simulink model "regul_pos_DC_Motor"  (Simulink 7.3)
settings: Solver=ode15s  StartTime=0.0  StopTime=150  RelTol=1e-3
StopFcn:
  | close all, clc
  | load pos_vit.mat
  | plot(x(1,:),x(2,:), x(1,:),x(4,:))
  | grid
  | title('Régulation de vitesse DC Motor')
  | gtext('Consigne)')
  | gtext('Position')
  | xlabel('temps')
  | figure
  | plotyy(x(1,:),x(3,:),x(1,:),x(5,:))
  | title('Position et Signal de commande')
  | gtext('signal de commande')
  | gtext('position linéaire')
  | grid
  | xlabel('temps')
libraries: fl_lib x17, nesl_utility x6, elec_lib x1

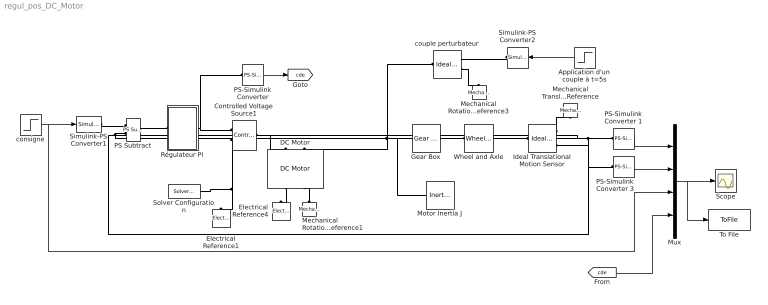
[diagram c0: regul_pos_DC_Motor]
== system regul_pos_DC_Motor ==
  Application d'un couple à t=5s : Step  Time=55  After=-0.5e-3  SampleTime=0
  Controlled Voltage Source1 : fl_lib/Electrical/Electrical Sources/Controlled Voltage Source  DialogController=NetworkEngine.DynNeDlgSource  SystemSampleTime=-1  i_Log=off  v_Log=off  LocalVarNames=|current|voltage|power  LocalVarDescs=|Current (A)|Voltage (V)|Power (W)  LocalVarLogging=[0 0 0]
  DC Motor : elec_lib/Actuators & Drivers/DC Motor  DialogController=NetworkEngine.DynNeDlgSource  SystemSampleTime=-1  parameterization=1  Ra=3.9 Ohm  La=1.2e-05 H  emf_or_torque=1  Kv=7.2e-05 V/rpm  Ki=6.876e-04 N*m/A  T_stall=2.4e-04 N*m  w_max=1.91e+04 rpm  w_rated=1.5e+04 rpm  P_rated=0.08 W  V_rated=1.5 V  J=0.01 g*cm^2  lam=1e-08 N*m/(rad/s)  speed0=0 rpm  current_Log=off  voltage_Log=off  power_Log=off  i2r_Log=off  torque_Log=off  speed_Log=off  LocalVarNames=|current|voltage|power|i2r|torque|speed  LocalVarDescs=|Current (A)|Voltage (V)|Power (W)|Electrical losses (W)|Torque (Nm)|Angular speed (rad/s)  LocalVarLogging=[0 0 0 0 0 0]
  Electrical Reference1 : fl_lib/Electrical/Electrical Elements/Electrical Reference  DialogController=NetworkEngine.DynNeDlgSource  SystemSampleTime=-1  i_Log=off  LocalVarNames=|i  LocalVarDescs=|i  LocalVarLogging=[]
  Electrical Reference4 : fl_lib/Electrical/Electrical Elements/Electrical Reference  DialogController=NetworkEngine.DynNeDlgSource  SystemSampleTime=-1  i_Log=off  LocalVarNames=|i  LocalVarDescs=|i  LocalVarLogging=[]
  Gear Box : fl_lib/Mechanical/Mechanisms/Gear Box  DialogController=NetworkEngine.DynNeDlgSource  SystemSampleTime=-1  ratio=5  t_in_Log=off  t_out_Log=off  LocalVarNames=|t_in|t_out  LocalVarDescs=|t_in|t_out  LocalVarLogging=[0 0]
  Ideal Translational Motion Sensor : fl_lib/Mechanical/Mechanical Sensors/Ideal Translational Motion Sensor  DialogController=NetworkEngine.DynNeDlgSource  SystemSampleTime=-1  offset=0 m  v_Log=off  f_Log=off  x_Log=off  LocalVarNames=|v|f|x  LocalVarDescs=|v|f|x  LocalVarLogging=[0 0 0]
  Mechanical Rotational Reference1 : fl_lib/Mechanical/Rotational Elements/Mechanical Rotational Reference  DialogController=NetworkEngine.DynNeDlgSource  SystemSampleTime=-1  t_Log=off  LocalVarNames=|t  LocalVarDescs=|t  LocalVarLogging=[]
  Mechanical Rotational Reference3 : fl_lib/Mechanical/Rotational Elements/Mechanical Rotational Reference  DialogController=NetworkEngine.DynNeDlgSource  SystemSampleTime=-1  t_Log=off  LocalVarNames=|t  LocalVarDescs=|t  LocalVarLogging=[]
  Mechanical Translational Reference : fl_lib/Mechanical/Translational Elements/Mechanical Translational Reference  DialogController=NetworkEngine.DynNeDlgSource  SystemSampleTime=-1  f_Log=off  LocalVarNames=|f  LocalVarDescs=|f  LocalVarLogging=0
  Motor Inertia J : fl_lib/Mechanical/Rotational Elements/Inertia  DialogController=NetworkEngine.DynNeDlgSource  SystemSampleTime=-1  inertia=10 g*cm^2  initial_velocity=0 rad/s  t_Log=off  LocalVarNames=|torque|velocity  LocalVarDescs=|Inertia torque (N*m)|Inertia absolute velocity (rad/s)  LocalVarLogging=[0 0]
  Mux : Mux
  PS Subtract : fl_lib/Physical Signals/Functions/PS Subtract  DialogController=NetworkEngine.DynNeDlgSource  SystemSampleTime=-1  LocalVarLogging=[]
  PS-Simulink Converter : nesl_utility/PS-Simulink Converter  DialogController=NetworkEngine.DynNeUtilDlgSource  SystemSampleTime=-1  PhysicalDomain=network_engine_domain  LeftPortType=input  RightPortType=output  SubClassName=ps_output  Unit=1  AffineConversion=off
  PS-Simulink Converter 1 : nesl_utility/PS-Simulink Converter  DialogController=NetworkEngine.DynNeUtilDlgSource  SystemSampleTime=-1  PhysicalDomain=network_engine_domain  LeftPortType=input  RightPortType=output  SubClassName=ps_output  Unit=1  AffineConversion=off
  PS-Simulink Converter 3 : nesl_utility/PS-Simulink Converter  DialogController=NetworkEngine.DynNeUtilDlgSource  SystemSampleTime=-1  PhysicalDomain=network_engine_domain  LeftPortType=input  RightPortType=output  SubClassName=ps_output  Unit=1  AffineConversion=off
  Régulateur PI : Subsystem
  Scope : Scope
  Simulink-PS Converter1 : nesl_utility/Simulink-PS Converter  DialogController=NetworkEngine.DynNeUtilDlgSource  SystemSampleTime=-1  PhysicalDomain=network_engine_domain  LeftPortType=input  RightPortType=output  SubClassName=ps_input  Unit=1  AffineConversion=off  InputFilterTimeConstant=.001  UdotUserProvided=0
  Simulink-PS Converter2 : nesl_utility/Simulink-PS Converter  DialogController=NetworkEngine.DynNeUtilDlgSource  SystemSampleTime=-1  PhysicalDomain=network_engine_domain  LeftPortType=input  RightPortType=output  SubClassName=ps_input  Unit=1  AffineConversion=off  InputFilterTimeConstant=.001  UdotUserProvided=0
  Solver Configuration : nesl_utility/Solver Configuration  DialogController=NetworkEngine.DynNeUtilDlgSource  SystemSampleTime=-1  PhysicalDomain=network_engine_domain  LeftPortType=input  RightPortType=generic  SubClassName=solver  Accelerate=off  Profile=off  ResidualTolerance=1e-9  MaxNonlinIter=12  MaxModeIter=2  DoFixedCost=off  DoDC=off  LinearAlgebra=Full
  To File : ToFile  Filename=pos_vit.mat  MatrixName=x
  Wheel and Axle : fl_lib/Mechanical/Mechanisms/Wheel and Axle  DialogController=NetworkEngine.DynNeDlgSource  SystemSampleTime=-1  R=0.05 m  or=1  torque_A_Log=off  force_P_Log=off  ang_velocity_Log=off  velocity_Log=off  LocalVarNames=|torque_A|force_P|ang_velocity|velocity  LocalVarDescs=|Axle torque (N*m)|Periphery force (N)|Axle angular velocity (rad/s)|Periphery velocity (m/s)  LocalVarLogging=[0 0 0 0]
  consigne : Step  Time=10  After=0.5  SampleTime=0
  couple perturbateur : fl_lib/Mechanical/Mechanical Sources/Ideal Torque Source  DialogController=NetworkEngine.DynNeDlgSource  SystemSampleTime=-1  w_Log=off  t_Log=off  LocalVarNames=|torque|rel_velocity|power  LocalVarDescs=|Torque (N*m)|Relative velocity (rad/s)|Power generated by the source (W)  LocalVarLogging=[0 0 0]
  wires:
  PS-Simulink Converter 1/1 -> Mux/1
  PS-Simulink Converter 3/1 -> Mux/2
  Mux/1 -> To File/1, Scope/1
  consigne/1 -> Simulink-PS Converter1/1, Mux/3
  Application d'un couple à t=5s/1 -> Simulink-PS Converter2/1
  PS-Simulink Converter/1 -> [cde]
  [cde] -> Mux/4
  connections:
  Ideal Translational Motion Sensor/RConn1 -- Mechanical Translational Reference/LConn1
  PS Subtract/LConn2 -- Ideal Translational Motion Sensor/RConn2 -- PS-Simulink Converter 1/LConn1
  Simulink-PS Converter1/RConn1 -- PS Subtract/LConn1
  Mechanical Rotational Reference1/LConn1 -- DC Motor/RConn2
  Motor Inertia J/LConn1 -- DC Motor/LConn2 -- Gear Box/LConn1 -- couple perturbateur/LConn1
  Wheel and Axle/LConn1 -- Gear Box/RConn1
  Wheel and Axle/RConn1 -- Ideal Translational Motion Sensor/LConn1
  DC Motor/RConn1 -- Electrical Reference4/LConn1
  Controlled Voltage Source1/LConn1 -- DC Motor/LConn1
  Controlled Voltage Source1/RConn2 -- Electrical Reference1/LConn1 -- Solver Configuration/RConn1
  Régulateur PI/RConn1 -- Controlled Voltage Source1/RConn1 -- PS-Simulink Converter/LConn1
  PS Subtract/RConn1 -- Régulateur PI/LConn1
  PS-Simulink Converter 3/LConn1 -- Ideal Translational Motion Sensor/RConn3
  couple perturbateur/RConn2 -- Mechanical Rotational Reference3/LConn1
  Simulink-PS Converter2/RConn1 -- couple perturbateur/RConn1

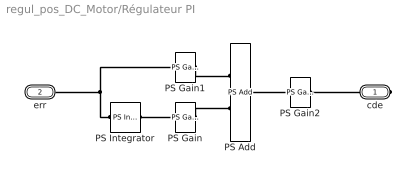
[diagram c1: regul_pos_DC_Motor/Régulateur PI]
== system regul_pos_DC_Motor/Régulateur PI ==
  PS Add : fl_lib/Physical Signals/Functions/PS Add  DialogController=NetworkEngine.DynNeDlgSource  SystemSampleTime=-1  LocalVarLogging=[]
  PS Gain : fl_lib/Physical Signals/Functions/PS Gain  DialogController=NetworkEngine.DynNeDlgSource  SystemSampleTime=-1  gain=0.1  LocalVarLogging=[]
  PS Gain1 : fl_lib/Physical Signals/Functions/PS Gain  DialogController=NetworkEngine.DynNeDlgSource  SystemSampleTime=-1  gain=1  LocalVarLogging=[]
  PS Gain2 : fl_lib/Physical Signals/Functions/PS Gain  DialogController=NetworkEngine.DynNeDlgSource  SystemSampleTime=-1  gain=0.8  LocalVarLogging=[]
  PS Integrator : fl_lib/Physical Signals/Linear Operators/PS Integrator  DialogController=NetworkEngine.DynNeDlgSource  SystemSampleTime=-1  x0=0  x_Log=off  LocalVarNames=|x  LocalVarDescs=|x  LocalVarLogging=0
  cde : PMIOPort  Port=1  Side=Right
  err : PMIOPort  Port=2  Side=Left
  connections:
  PS Gain1/RConn1 -- PS Add/LConn1
  PS Gain/RConn1 -- PS Add/LConn2
  PS Integrator/RConn1 -- PS Gain/LConn1
  PS Gain1/LConn1 -- PS Integrator/LConn1 -- err/RConn1
  PS Gain2/RConn1 -- cde/RConn1
  PS Add/RConn1 -- PS Gain2/LConn1
